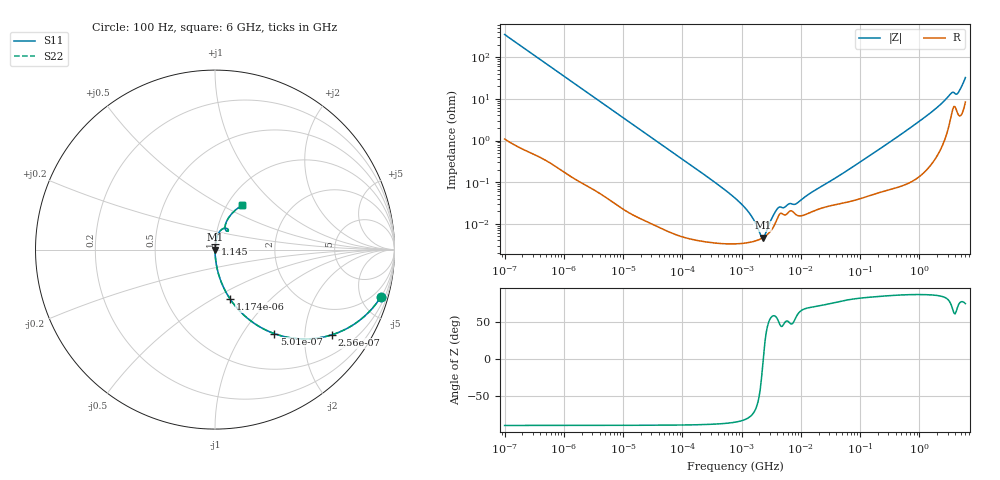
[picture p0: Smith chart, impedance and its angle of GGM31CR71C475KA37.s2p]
!Murata Part Number: GGM31CR71C475KA37
!These Parameters are Measured in Series Mode Connection
!Data Generated on Jun 19, 2026
!  o--ll--o
!Port1  Port2
!  o------o
!Operation Temp=25[degC], DC Bias Voltage=0[V]
!Freq. Start=100[Hz] Stop=6[GHz] 401[Steps]
# Hz S RI R 50
!Freq.(Hz) S11(Real) S11(Imag) S21(Real) S21(Imag) S12(Real) S12(Imag) S22(Real) S22(Imag)
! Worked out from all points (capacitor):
!   401 points, 100 Hz to 6 GHz, reference 50 ohm
!   read as one part in series: C = 4.53 uF near 109 Hz
!   lowest |Z| = 4.68 mohm at 2.269 MHz (marker M1)
!   series resonance near 2.322 MHz, so ESL is about 1 nH
!   S11 on the Smith chart (normalised r, x): 100 Hz: 1.02, -7.02; 256 Hz: 1.01, -2.75; 501 Hz: 1.01, -1.41; 1.174 kHz: 1.00, -0.60; 1.145 GHz: 1.00, +0.07; 6 GHz: 1.17, +0.63
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100  0.9242 -0.2632  0.0758 0.2632  0.0758 0.2632  0.9242 -0.2632
164  0.8208 -0.3819  0.1792 0.3819  0.1792 0.3819  0.8208 -0.3819
256  0.6527 -0.4742  0.3473 0.4742  0.3473 0.4742  0.6527 -0.4742
501  0.3313 -0.4683  0.6687 0.4683  0.6687 0.4683  0.3313 -0.4683
750  0.1823 -0.3836  0.8177 0.3836  0.8177 0.3836  0.1823 -0.3836
1174  0.0842 -0.2752  0.9158 0.2752  0.9158 0.2752  0.0842 -0.2752
2008  0.031 -0.1705  0.969 0.1705  0.969 0.1705  0.031 -0.1705
6433  0.00338 -0.055  0.9966 0.055  0.9966 0.055  0.00338 -0.055
40335  0.000161 -0.00886  0.9998 0.00886  0.9998 0.00886  0.000161 -0.00886
774597  3.34e-05 -0.000416  1 0.000416  1 0.000416  3.34e-05 -0.000416
1212075  3.5e-05 -0.000219  1 0.000219  1 0.000219  3.5e-05 -0.000219
1734173  3.92e-05 -9.38e-05  1 9.38e-05  1 9.38e-05  3.92e-05 -9.38e-05
2268635  4.62e-05 -7.4e-06  1 7.4e-06  1 7.4e-06  4.62e-05 -7.4e-06
2967816  6.26e-05 8.28e-05  0.9999 -8.28e-05  0.9999 -8.28e-05  6.26e-05 8.28e-05
4246196  0.00016 0.000192  0.9998 -0.000192  0.9998 -0.000192  0.00016 0.000192
8311524  0.000166 0.000254  0.9998 -0.000254  0.9998 -0.000254  0.000166 0.000254
1.555665e7  0.000197 0.00055  0.9998 -0.00055  0.9998 -0.00055  0.000197 0.00055
3.124326e8  0.000741 0.009  0.9993 -0.009  0.9993 -0.009  0.000741 0.009
1.144649e9  0.0027 0.0332  0.9973 -0.0332  0.9973 -0.0332  0.0027 0.0332
3.352442e9  0.0456 0.117  0.9544 -0.117  0.9544 -0.117  0.0456 0.117
4.385646e9  0.058 0.1114  0.942 -0.1114  0.942 -0.1114  0.058 0.1114
6e9  0.1488 0.2461  0.8512 -0.2461  0.8512 -0.2461  0.1488 0.2461
